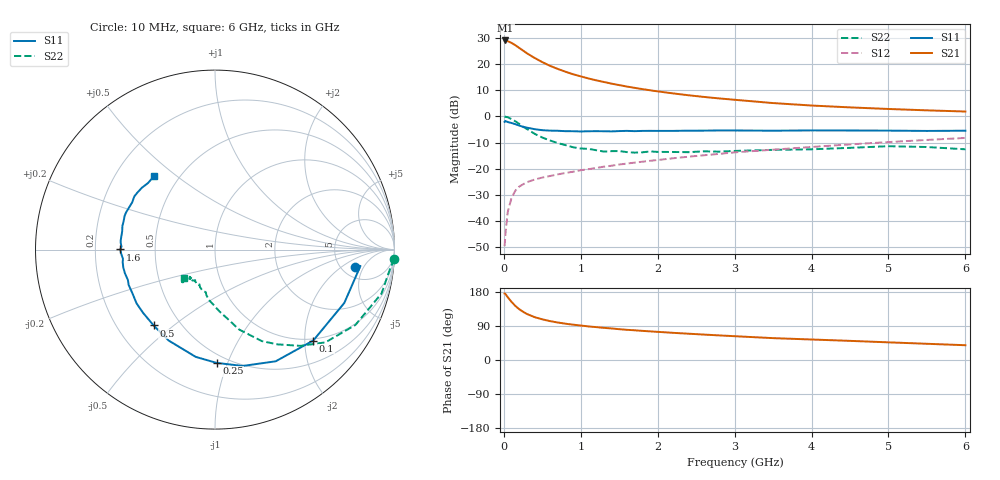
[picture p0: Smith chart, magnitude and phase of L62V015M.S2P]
!  INFINEON TECHNOLOGIES Small Signal Semiconductors
! BFR380L3 , Si-NPN RF-Transistor in TSLP-3-1
!  Vce=2 V,  Ic=15 mA
! Common Emitter S-Parameters:  07. March 2005
#  GHz  S  MA  R  50
! f  S11  S21  S12  S22
! GHz  Mag  Ang  Mag  Ang  Mag  Ang  Mag  Ang
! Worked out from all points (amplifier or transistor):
!   36 points, 10 MHz to 6 GHz, reference 50 ohm
!   highest |S21| = 29.0 dB at 20 MHz (marker M1)
!   |S21| within 3 dB of that: start of sweep to 207.1 MHz
!   unconditionally stable (mu >= 1): 1.962 GHz to 4.846 GHz
!   at 250 MHz: K = 0.32, MSG = 25.6 dB, |S12| = -26.0 dB
!   at 1.4 GHz: K = 0.93, MSG = 15.7 dB, |S12| = -18.9 dB
!   at 6 GHz: K = 0.97, MSG = 5.0 dB, |S12| = -8.3 dB
!   S11 on the Smith chart (normalised r, x): 10 MHz: 6.61, -3.29; 100 MHz: 0.96, -2.19; 250 MHz: 0.44, -0.91; 500 MHz: 0.36, -0.43; 1.6 GHz: 0.31, +0.00; 6 GHz: 0.37, +0.42
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0.01  0.7844 -7.0  28.2 175.3  0.0033 85.9  1.001 -3.0
0.02  0.8154 -6.4  28.21 174.5  0.0054 82.1  0.9818 -6.1
0.05  0.7794 -22.4  27.36 165.9  0.0147 82.2  0.9597 -14.7
0.1  0.7459 -42.8  25.32 153.4  0.0277 70.7  0.8881 -28.2
0.15  0.7082 -61.5  22.86 142.6  0.038 63.1  0.8037 -40.0
0.2  0.6664 -76.6  20.3 134.0  0.0454 58.8  0.7172 -48.4
0.25  0.6313 -89.2  18.07 127.3  0.0503 53.9  0.6324 -56.6
0.3  0.6072 -100.2  16.05 121.5  0.0551 52.0  0.5728 -62.9
0.4  0.5686 -117.1  13.05 113.1  0.0621 49.3  0.4643 -73.3
0.5  0.5436 -129.0  10.88 107.3  0.0676 48.8  0.3933 -79.5
0.6  0.5336 -138.7  9.242 102.6  0.0724 48.8  0.3461 -85.8
0.7  0.5299 -145.5  8.068 99.0  0.0777 50.2  0.3085 -91.4
0.9  0.5197 -157.8  6.381 93.2  0.0873 52.2  0.2568 -100.9
1.1  0.519 -165.3  5.303 88.6  0.0979 54.2  0.2392 -107.0
1.4  0.5154 -174.3  4.217 83.3  0.1138 56.3  0.2163 -114.4
1.6  0.5276 179.9  3.712 79.7  0.125 57.5  0.2073 -122.5
2.2  0.5271 168.9  2.746 71.7  0.158 60.0  0.2084 -126.9
2.8  0.5376 159.4  2.2 64.9  0.1918 61.3  0.2114 -133.9
3.5  0.5312 150.3  1.793 57.7  0.2307 60.5  0.2288 -134.1
4.5  0.5365 143.6  1.483 50.5  0.2909 60.0  0.25 -134.5
5.5  0.5262 135.2  1.302 42.8  0.3539 57.1  0.2592 -135.0
6  0.5314 129.9  1.236 39.0  0.3868 55.3  0.2344 -137.3
